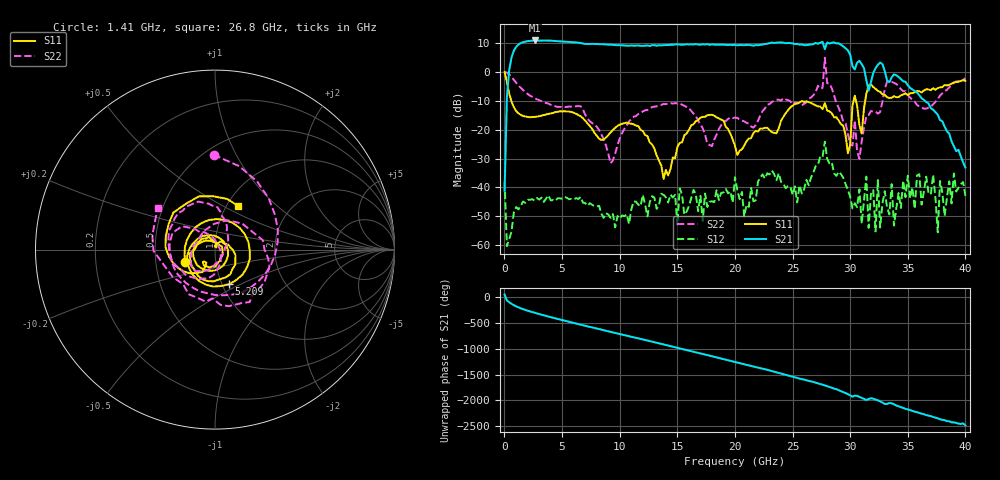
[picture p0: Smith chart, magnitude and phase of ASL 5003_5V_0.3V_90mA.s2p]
!ASL 5003 Ultra Wideband Amplifier
!Test Fixture S-parameter data in 10MHz-40GHz
!Bias Conditions Vdd=5V,Vg = -0.3V,; Ids =90mA
!Agilent Technologies,N5230A,MY45000142,A.04.83
!Agilent N5230A: A.04.83
!Date: Friday, September 08, 2006 16:40:49
!Correction: S11(Full 2 Port SOLT,1,2) S21(Full 2 Port SOLT,1,2) S12(Full 2 Port SOLT,1,2) S22(Full 2 Port SOLT,1,2)
!S2P File: Measurements: S11, S21, S12, S22:
# Hz S  dB  R 50
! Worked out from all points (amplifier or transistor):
!   201 points, 10 MHz to 40 GHz, reference 50 ohm
!   highest |S21| = 10.8 dB at 2.609 GHz (marker M1)
!   |S21| within 3 dB of that: 891.2 MHz to 27.8 GHz (26.91 GHz wide, 188 % of centre)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
!   unconditionally stable (mu >= 1): start of sweep to 27.71 GHz; 27.91 GHz to end of sweep
!   at 6.608 GHz: K = 21.01, MAG = 10.4 dB, |S12| = -43.3 dB
!   at 20 GHz: K = 11.01, MAG = 9.5 dB, |S12| = -36.5 dB
!   at 40 GHz: K = 640.63, MAG = -26.2 dB, |S12| = -42.9 dB
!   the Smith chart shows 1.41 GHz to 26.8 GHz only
!   S11 on the Smith chart (normalised r, x): 1.41 GHz: 0.71, -0.10; 5.209 GHz: 1.08, -0.44; 26.8 GHz: 1.13, +0.59
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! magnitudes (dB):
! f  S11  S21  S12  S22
! 10 MHz  -0.1  -41.2  -38.0  -0.1
! 209.9 MHz  -3.5  -8.7  -60.3  -0.3
! 409.9 MHz  -7.5  0.6  -57.9  -0.9
! 1.41 GHz  -14.9  9.9  -46.4  -5.5
! 2.609 GHz  -15.6  10.8  -44.6  -9.1
! 5.209 GHz  -13.6  10.4  -43.2  -12.2
! 6.808 GHz  -16.0  9.8  -45.3  -13.0
! 9.208 GHz  -21.0  9.4  -50.5  -31.7
! 13.41 GHz  -30.6  9.2  -46.1  -11.7
! 17.61 GHz  -15.0  9.6  -46.8  -24.9
! 20 GHz  -25.6  9.4  -36.5  -15.9
! 20.8 GHz  -25.5  9.2  -50.1  -17.1
! 26.8 GHz  -11.2  9.6  -34.8  -8.1
! 27.8 GHz  -10.8  7.8  -24.1  4.9
! 29.8 GHz  -28.2  7.4  -40.9  -21.5
! 30.4 GHz  -8.3  0.8  -45.5  -16.8
! 30.8 GHz  -18.4  3.8  -40.7  -30.1
! 33.4 GHz  -9.1  -3.6  -49.3  -3.5
! 35 GHz  -8.0  -4.6  -35.9  -8.0
! 37.2 GHz  -5.7  -13.1  -35.6  -11.2
! 37.6 GHz  -5.6  -14.8  -55.5  -9.4
! 40 GHz  -3.1  -33.1  -42.9  -2.2
